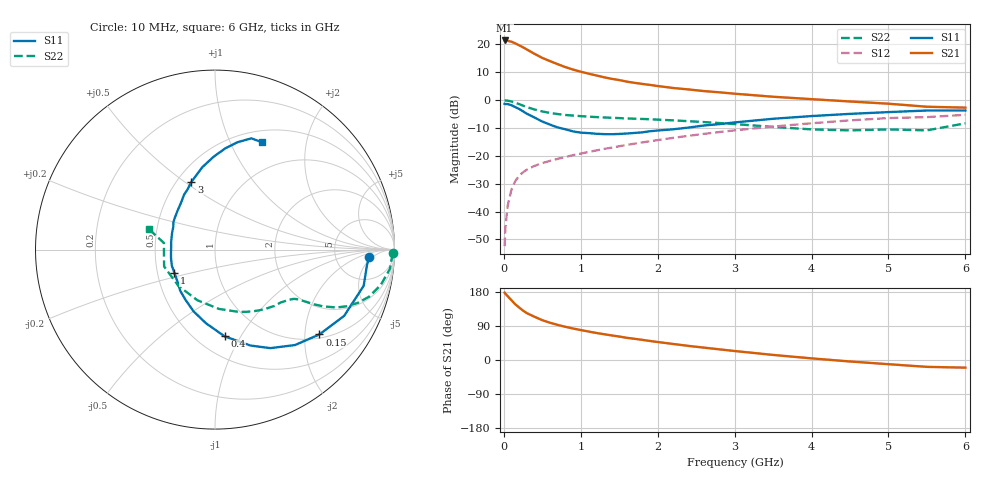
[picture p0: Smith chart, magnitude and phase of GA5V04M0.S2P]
! Infineon Technologies  Discrete & RF Semiconductors
! BF775
! Si NPN RF Bipolar Junction Transistor in SOT23
! VCE = 5 V  IC = 4 mA
! Common Emitter S-Parameters:  May  1996
# GHz  S  MA  R  50
!  f  S11  S21  S12  S22
! GHz  MAG  ANG  MAG  ANG  MAG  ANG  MAG  ANG
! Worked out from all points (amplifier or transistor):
!   36 points, 10 MHz to 6 GHz, reference 50 ohm
!   highest |S21| = 21.4 dB at 10 MHz (marker M1)
!   |S21| within 3 dB of that: start of sweep to 283.8 MHz
!   unconditionally stable (mu >= 1): 894.5 MHz to 3.289 GHz
!   at 250 MHz: K = 0.42, MSG = 22.4 dB, |S12| = -25.9 dB
!   at 1.4 GHz: K = 1.12, MAG = 10.3 dB, |S12| = -17.0 dB
!   at 6 GHz: K = 0.94, MSG = 1.3 dB, |S12| = -5.3 dB
!   S11 on the Smith chart (normalised r, x): 10 MHz: 12, -4; 150 MHz: 1.10, -2.37; 400 MHz: 0.68, -0.86; 1 GHz: 0.61, -0.17; 3 GHz: 0.59, +0.53; 6 GHz: 0.64, +1.32
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0.01  0.8601 -2.8  11.79 177.6  0.0024 88.1  0.9946 -1.2
0.02  0.8514 -5.6  11.75 174.9  0.0051 86.1  0.9865 -2.6
0.05  0.8526 -13.7  11.6 168.4  0.0128 83.0  0.9804 -6.3
0.1  0.8089 -27.1  11.19 157.5  0.0251 76.2  0.9447 -12.0
0.15  0.7494 -39.1  10.42 146.7  0.0356 69.6  0.8976 -17.0
0.2  0.694 -50.0  9.633 138.3  0.0442 65.6  0.8488 -20.5
0.25  0.6295 -60.7  8.871 130.2  0.0508 61.5  0.7959 -23.4
0.3  0.5699 -69.7  8.104 123.6  0.0567 59.1  0.7493 -25.5
0.4  0.4862 -83.7  6.765 113.9  0.0662 56.1  0.6801 -27.7
0.5  0.4133 -97.0  5.733 105.1  0.0742 54.7  0.6276 -29.0
0.6  0.3641 -109.2  5.017 98.3  0.0815 54.3  0.5898 -29.7
0.7  0.3242 -120.5  4.422 92.6  0.0884 54.6  0.5638 -30.3
0.8  0.3003 -130.2  3.919 87.6  0.0956 54.7  0.5425 -30.8
1  0.2614 -149.7  3.242 79.0  0.1101 55.1  0.5168 -32.1
1.1  0.2565 -159.8  2.996 75.2  0.1177 55.7  0.5066 -33.2
1.6  0.2523 163.0  2.15 58.5  0.1578 56.0  0.4694 -39.0
2.2  0.3002 134.2  1.654 42.3  0.2104 53.7  0.4344 -49.4
3  0.3986 109.4  1.306 23.7  0.2874 47.5  0.3727 -68.8
3.5  0.4638 98.9  1.152 13.4  0.3357 42.2  0.3313 -86.1
4.5  0.5677 84.1  0.947 -3.9  0.4341 29.9  0.2871 -135.3
5.5  0.6521 71.9  0.762 -18.1  0.4964 14.5  0.2874 172.5
6  0.6528 66.4  0.735 -20.2  0.5453 10.3  0.3843 162.9
